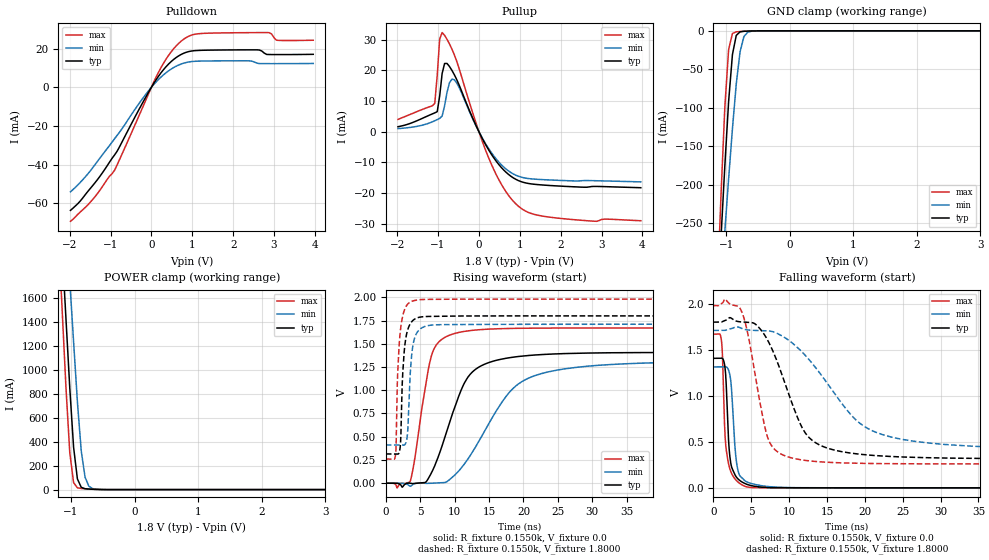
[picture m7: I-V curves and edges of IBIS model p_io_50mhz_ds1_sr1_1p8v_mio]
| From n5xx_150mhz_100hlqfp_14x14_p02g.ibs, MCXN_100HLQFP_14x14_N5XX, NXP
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[Model] p_io_50mhz_ds1_sr1_1p8v_mio
|   Model p_io_50mhz_ds1_sr1_1p8v_mio
| This model was characterised for following simulation conditions:
| External (pad) voltage:
|   - Typ: 1.8V,   - Min: 1.71V,   - Max: 1.98V
| Library cells for typ/min/max conditions are connected as defined below:
|  pad - External Pad
|  ipp_do_lv - Core Input
|  ipp_obe_lv - Output Buffer Enable
|  IOGC - NC
|  REFH3V3 - REFH3V3
|  REFL3V3 - REFL3V3
|  ZI - NC
|  abut_ncal_vddio[1] - vssio vddio vddio
|  abut_ncal_vddio[2] - vddio vddio vssio
|  abut_ncal_vddio[3] - vddio
|  abut_ncal_vddio[4] - vssio vddio vddio
|  abut_ncal_vddio[5] - vddio vddio vssio
|  abut_ncal_vddio[6] - vddio
|  abut_pcal_vddio[1] - vssio
|  abut_pcal_vddio[2] - vddio vssio vddio
|  abut_pcal_vddio[3] - vssio
|  abut_pcal_vddio[4] - vssio
|  abut_pcal_vddio[5] - vddio vssio vddio
|  abut_pcal_vddio[6] - vssio
|  ipp_do_1p8v - ipp_do_1p8v
|  ipp_dse_lv - vdd_lv
|  ipp_eftd_lv - NC
|  ipp_ina_mux_vddio - NC
|  ipp_ina_mux_vddio[0] - NC
|  ipp_ina_mux_vddio[1] - NC
|  ipp_ina_r0_vddio - NC
|  ipp_ina_r0a_vddio - NC
|  ipp_ina_r0b_vddio - NC
|  ipp_ina_r0c_vddio - NC
|  ipp_ina_r0d_vddio - NC
|  ipp_ina_r0e_vddio - NC
|  ipp_ina_r0f_vddio - NC
|  ipp_ina_r300_vddio - NC
|  ipp_ina_r300a_vddio - NC
|  ipp_ina_r300b_vddio - NC
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Model_type I/O
Polarity   Non-Inverting
Enable   Active-High
Vinl =   0.5400V
Vinh =   1.2600V
Vmeas =  0.9000V
Cref =   30.0000pF
Rref =   1.0000M
Vref =   1.8000V
C_comp   1.4770pF   1.4118pF   1.5590pF
|C_comp_pullup   0.7610pF   0.7875pF   0.7350pF
|C_comp_pulldown   0.6300pF   0.6835pF   0.5882pF
[Model Spec]
| variable   typ   min   max
Vinh   1.2600V   1.1970V   1.3860V
Vinl   0.5400V   0.5130V   0.5940V
[Temperature Range]   25.0000   0.1250k   -40.0000
[Voltage Range]   1.8000V   1.7100V   1.9800V
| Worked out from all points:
|   slope of the pulldown table from 0 to 0.27 V, typ, clamps not added: 32.1 ohm
|   slope of the pullup table from 0 to 0.27 V, typ, clamps not added: 40.9 ohm
|   GND clamp passes 1 mA (typ) near -0.75 V on its own axis
|   POWER clamp passes 1 mA (typ) near -0.55 V on its own axis
|   rising waveform, R_fixture 0.1550k, V_fixture 0.0: 20-80 % time 4.19ns typ, 7.02ns min, 2.15ns max; typ from 0 V to 1.41 V
|   rising waveform, R_fixture 0.1550k, V_fixture 1.8000: 20-80 % time 568ps typ, 613ps min, 561ps max; typ from 0.315 V to 1.8 V
|   falling waveform, R_fixture 0.1550k, V_fixture 0.0: 20-80 % time 579ps typ, 667ps min, 606ps max; typ from 1.41 V to 0 V
|   falling waveform, R_fixture 0.1550k, V_fixture 1.8000: 20-80 % time 4.25ns typ, 7.85ns min, 2.32ns max; typ from 1.8 V to 0.315 V
[Pulldown]
|Voltage   I(typ)   I(min)   I(max)
-1.98V    -63.59mA   -54.01mA   -69.25mA
-1.44V    -50.89mA   -41.69mA   -58.07mA
-900mV    -34.94mA   -26.56mA   -42.81mA
180mV     5.908mA    4.185mA    8.001mA
480mV     13.23mA    9.376mA    18.23mA
780mV     17.5mA     12.4mA     24.7mA
1.2V      19.1mA     13.55mA    27.77mA
2.58V     19.36mA    12.5mA     28.27mA
2.82V     16.99mA    12.23mA    28.29mA
2.94V     16.93mA    12.23mA    27.6mA
3.06V     16.92mA    12.23mA    24.35mA
3.96V     17.05mA    12.32mA    24.33mA
[Pullup]
|Voltage   I(typ)   I(min)   I(max)
-1.98V    1.62mA     998.6uA    4.005mA
-1.08V    6.133mA    3.566mA    9.235mA
-1.02V    6.531mA    3.947mA    18.33mA
-960mV    11.63mA    4.346mA    30.19mA
-900mV    18.95mA    5.088mA    32.31mA
-840mV    22.23mA    8.438mA    31.4mA
-720mV    21.25mA    15.95mA    28.6mA
-600mV    18.53mA    16.91mA    25.01mA
240mV     -5.967mA   -5.552mA   -8.574mA
900mV     -15.51mA   -14.17mA   -23.49mA
1.68V     -17.49mA   -15.7mA    -27.77mA
3.96V     -18.27mA   -16.36mA   -29.03mA
[GND_clamp]
|Voltage   I(typ)   I(min)   I(max)
-1.98V    -1.861A    -1.524A    -2.333A
-1.14V    -366mA     -404.8mA   -340.6mA
-1.08V    -268.7mA   -331.9mA   -213.6mA
-1.02V    -175.9mA   -260.7mA   -99.61mA
-960mV    -91.54mA   -192mA     -24.26mA
-900mV    -30.77mA   -127.1mA   -3.42mA
-840mV    -5.96mA    -68.91mA   -1.328mA
-780mV    -1.308mA   -27.16mA   -908.9uA
-720mV    -590.1uA   -7.523mA   -630.1uA
-660mV    -358.7uA   -1.802mA   -403.9uA
-420mV    -15.5uA    -34.2uA    -9.716uA
3.96V     0A         0A         0A
[POWER_clamp]
|Voltage   I(typ)   I(min)   I(max)
-1.98V    10.29A     9.986A     10.79A
-1.2V     2.598A     3.277A     2.158A
-1.14V    2.012A     2.764A     1.504A
-1.08V    1.429A     2.253A     855.2mA
-1.02V    851mA      1.743A     310.4mA
-960mV    354.2mA    1.236A     58.61mA
-900mV    89.61mA    734.2mA    15.24mA
-840mV    19.5mA     326mA      9.554mA
-780mV    7.508mA    104.4mA    6.926mA
-720mV    4.523mA    28.33mA    4.778mA
-660mV    2.875mA    8.601mA    2.988mA
3.96V     0A         0A         0A
[Ramp]
| variable   typ   min   max
dV/dt_r  0.8441/4.1915n   0.7880/7.0237n   1.0018/2.1453n
dV/dt_f  0.8911/4.2468n   0.7793/7.8523n   1.0321/2.3173n
R_load = 0.1550k
[Rising Waveform]
R_fixture= 0.1550k
V_fixture= 0.0
V_fixture_min= 0.0
V_fixture_max= 0.0
|time   V(typ)   V(min)   V(max)
0s        513.4pV    165.8nV    14.19pV
3.546ns   -178.9uV   -33.27mV   22.13mV
6.065ns   37.15mV    -1.775mV   1.181V
7.169ns   199.4mV    1.518mV    1.468V
10.94ns   1.001V     161.6mV    1.627V
12.86ns   1.215V     368.1mV    1.647V
16.96ns   1.337V     882.1mV    1.663V
19.81ns   1.367V     1.095V     1.667V
32.35ns   1.403V     1.275V     1.67V
235ns     1.407V     1.313V     1.67V
[Rising Waveform]
R_fixture= 0.1550k
V_fixture= 1.8000
V_fixture_min= 1.7100
V_fixture_max= 1.9800
|time   V(typ)   V(min)   V(max)
0s        314.8mV    411.2mV    259.8mV
1.414ns   315.2mV    411.1mV    309.9mV
1.687ns   313.2mV    411.1mV    1.123V
2.035ns   360.4mV    411.4mV    1.583V
2.438ns   1.162V     410mV      1.795V
2.948ns   1.58V      442.1mV    1.903V
3.179ns   1.651V     562.1mV    1.927V
3.786ns   1.739V     1.403V     1.957V
4.858ns   1.785V     1.651V     1.974V
235ns     1.8V       1.71V      1.98V
[Falling Waveform]
R_fixture= 0.1550k
V_fixture= 0.0
V_fixture_min= 0.0
V_fixture_max= 0.0
|time   V(typ)   V(min)   V(max)
0s        1.407V     1.313V     1.67V
1.073ns   1.409V     1.313V     1.596V
1.209ns   1.406V     1.313V     1.42V
1.559ns   1.291V     1.316V     548.2mV
2.055ns   454.1mV    1.267V     242.6mV
2.363ns   242mV      1.109V     164.7mV
2.823ns   147.3mV    474.6mV    100.9mV
3.169ns   104.2mV    220.8mV    69.43mV
4.846ns   27.47mV    51.27mV    5.161mV
235ns     1.094uV    2.269uV    699.3nV
[Falling Waveform]
R_fixture= 0.1550k
V_fixture= 1.8000
V_fixture_min= 1.7100
V_fixture_max= 1.9800
|time   V(typ)   V(min)   V(max)
0s        1.8V       1.71V      1.98V
1.55ns    1.818V     1.711V     2.05V
3.768ns   1.802V     1.73V      1.908V
6.834ns   1.651V     1.707V     648mV
7.657ns   1.524V     1.7V       462.1mV
11.36ns   716.4mV    1.505V     307.5mV
13.3ns    501mV      1.327V     287.9mV
20.88ns   353.9mV    624.4mV    264.7mV
34.29ns   320.2mV    452.2mV    260.1mV
235ns     314.8mV    411.2mV    259.8mV
